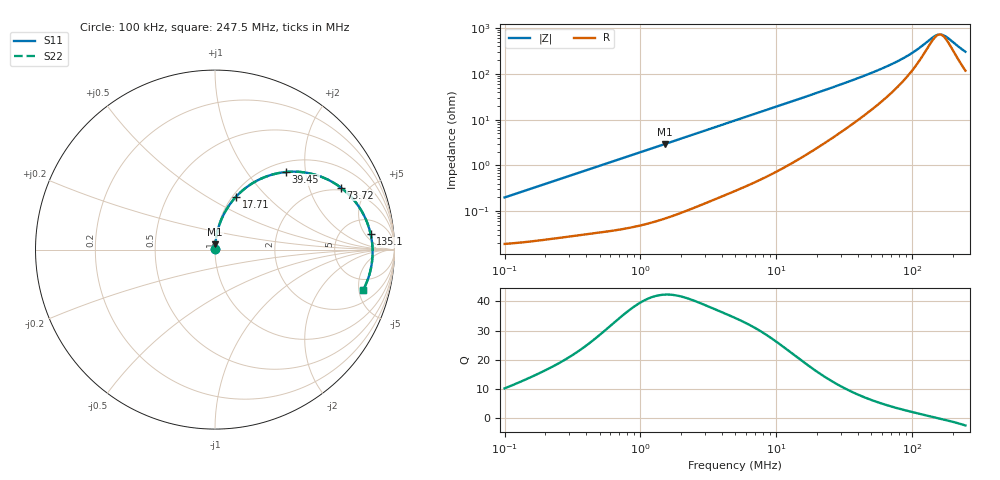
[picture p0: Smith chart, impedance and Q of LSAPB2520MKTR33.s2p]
! LSAPB2520MKTR33  S-PARAMETER MODEL  ( General Type )
! Model Generated by TAIYO YUDEN Corporation (http://www.ty-top.com)
! Version 3.0
! TAIYO YUDEN Control No. 20210629
! Copyright(c) 2015 TAIYO YUDEN CO.,LTD. All Rights Reserved.
! Product Description (link to TY-COMPAS)
! https://ds.yuden.co.jp/TYCOMPAS/or/detail?pn=LSAPB2520MKTR33M&u=M
! Products Name : Inductors
! Characteristics :
!  Inductance : 0.33 uH , SRF(min) : -Hz , DC Resistance(max) : 0.023 Ohm
!  Rated Current : Saturation :6600 mA , Temp Rise : 4400 mA (40 degC)
!  Case Size : 2.5 x 2.0 / 0.098 x 0.079 [mm/inch] , Thickness : 1.2 / 0.047 [mm/inch]
!  (Conditions: Temperature = 25 degC , DC Bias Current/Voltage = 0A / 0V)
! External Node Assignments :
!  1  o---GGG---o  2
! GND o---------o GND
! Frequency Range : 0.1MHz  -  247.502633MHz  [ 402 STEP ]
# MHz S RI R 50
! Freq[MHz].  S11 Real  S11 Imag  S21 Real  S21 Imag  S12 Real  S12 Imag  S22 Real  S22 Imag
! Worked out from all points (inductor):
!   401 points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, 100 kHz to 247.5 MHz, reference 50 ohm
!   read as one part in series: L = 317 nH near 104 kHz
!   highest Q = 42.3 at 1.511 MHz (marker M1), where L = 308 nH
!   self-resonance near 159.8 MHz
!   S11 on the Smith chart (normalised r, x): 100 kHz: 1.00, +0.00; 17.71 MHz: 1.04, +0.68; 39.45 MHz: 1.19, +1.57; 73.72 MHz: 1.87, +3.31; 135.1 MHz: 10, +7; 247.5 MHz: 3.34, -5.58
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0.1  0.000198 0.00199  0.9998 -0.00199  0.9998 -0.00199  0.000198 0.00199
0.37019  0.000357 0.00725  0.9996 -0.00725  0.9996 -0.00725  0.000357 0.00725
1.370406  0.00133 0.0265  0.9987 -0.0265  0.9987 -0.0265  0.00133 0.0265
1.511016  0.00154 0.0292  0.9985 -0.0292  0.9985 -0.0292  0.00154 0.0292
4.974964  0.0116 0.0937  0.9884 -0.0937  0.9884 -0.0937  0.0116 0.0937
10.45153  0.045 0.1886  0.955 -0.1886  0.955 -0.1886  0.045 0.1886
17.71114  0.1165 0.2937  0.8835 -0.2937  0.8835 -0.2937  0.1165 0.2937
18.41681  0.1246 0.3024  0.8754 -0.3024  0.8754 -0.3024  0.1246 0.3024
26.69375  0.2298 0.3819  0.7702 -0.3819  0.7702 -0.3819  0.2298 0.3819
39.45378  0.3962 0.4324  0.6038 -0.4324  0.6038 -0.4324  0.3962 0.4324
51.86374  0.5339 0.4234  0.4661 -0.4234  0.4661 -0.4234  0.5339 0.4234
68.1772  0.6671 0.3688  0.3329 -0.3688  0.3329 -0.3688  0.6671 0.3688
73.71824  0.7013 0.3453  0.2987 -0.3453  0.2987 -0.3453  0.7013 0.3453
100.767  0.8111 0.2245  0.1889 -0.2245  0.1889 -0.2245  0.8111 0.2245
115.5329  0.8433 0.1617  0.1567 -0.1617  0.1567 -0.1617  0.8433 0.1617
135.0757  0.8675 0.0854  0.1325 -0.0854  0.1325 -0.0854  0.8675 0.0854
151.8732  0.8765 0.026  0.1235 -0.026  0.1235 -0.026  0.8765 0.026
161.0397  0.8781 -0.00404  0.1219 0.00404  0.1219 0.00404  0.8781 -0.00404
167.456  0.878 -0.0242  0.122 0.0242  0.122 0.0242  0.878 -0.0242
181.0659  0.8752 -0.0646  0.1248 0.0646  0.1248 0.0646  0.8752 -0.0646
228.8991  0.8444 -0.1846  0.1556 0.1846  0.1556 0.1846  0.8444 -0.1846
247.5026  0.8264 -0.2232  0.1736 0.2232  0.1736 0.2232  0.8264 -0.2232
